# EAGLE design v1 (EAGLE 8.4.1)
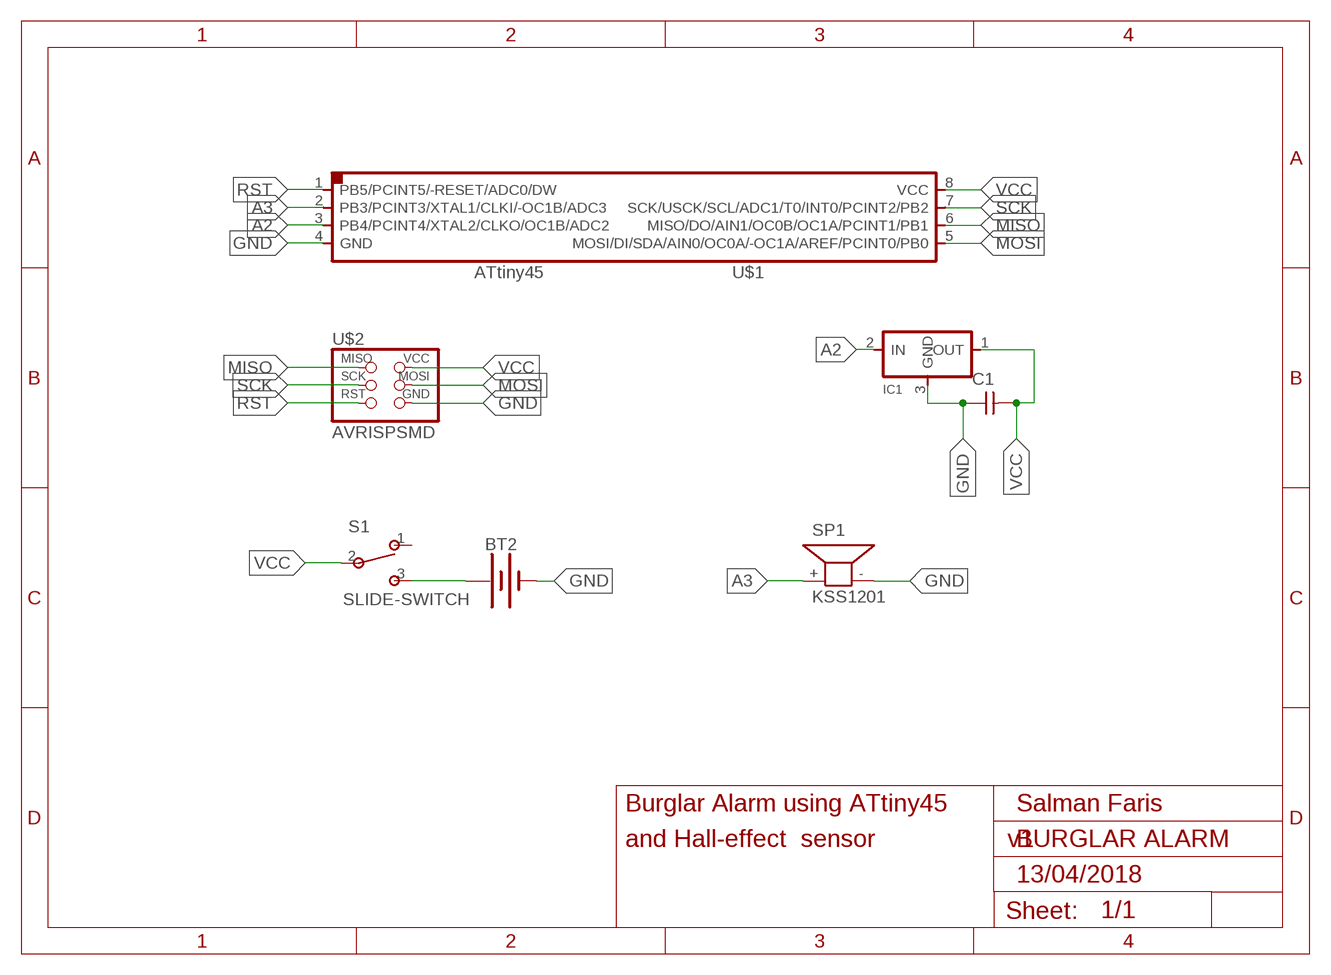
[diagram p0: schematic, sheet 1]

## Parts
BT2  BATTERY-20MM_PTH  [BATTCOM_20MM_PTH]
C1  CAP-UNPOLARIZEDFAB  [C1206FAB]
IC1  REGULATORSOT23  [SOT23]
S1  SLIDE-SWITCH  [AYZ0102AGRLC]
SP1  KSS1201  [KSS1201]
U$1  ATTINY45SI  [SOIC8]
U$2  AVRISPSMD  [2X03SMD]

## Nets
A2: IC1.2(IN) U$1.3(PB4/PCINT4/XTAL2/CLKO/OC1B/ADC2)
A3: SP1.+ U$1.2(PB3/PCINT3/XTAL1/CLKI/-OC1B/ADC3)
GND: BT2.2(-) C1.1 IC1.3(GND) SP1.- U$1.4(GND) U$2.6(GND)
MISO: U$1.6(MISO/DO/AIN1/OC0B/OC1A/PCINT1/PB1) U$2.1(MISO)
MOSI: U$1.5(MOSI/DI/SDA/AIN0/OC0A/-OC1A/AREF/PCINT0/PB0) U$2.4(MOSI)
N$1: BT2.1(+) S1.3
RST: U$1.1(PB5/PCINT5/-RESET/ADC0/DW) U$2.5(RST)
SCK: U$1.7(SCK/USCK/SCL/ADC1/T0/INT0/PCINT2/PB2) U$2.3(SCK)
VCC: C1.2 IC1.1(OUT) S1.2 U$1.8(VCC) U$2.2(VCC)
Unconnected: S1.1

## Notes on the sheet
- Burglar Alarm using ATtiny45 | Salman Faris
- and Hall-effect  sensor | BURGLAR ALARM
- 13/04/2018

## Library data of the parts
BT2 = SparkFun-Batteries:BATTERY: Battery - Single Cell; PROD_ID: BATT-09031; SF_SKU: PRT-00783
C1 = fab:CAP-UNPOLARIZED
IC1 = fab:REGULATOR
S1 = fab:SLIDE-SWITCH: SMD slide-switch AYZ0102AGRLC as found in the fablab inventory. Includes the mounting holes. Made by Zaerc.
SP1 = buzzer:KSS1201: SPEAKER
U$1 = fab:ATTINY45
U$2 = fab:AVRISP

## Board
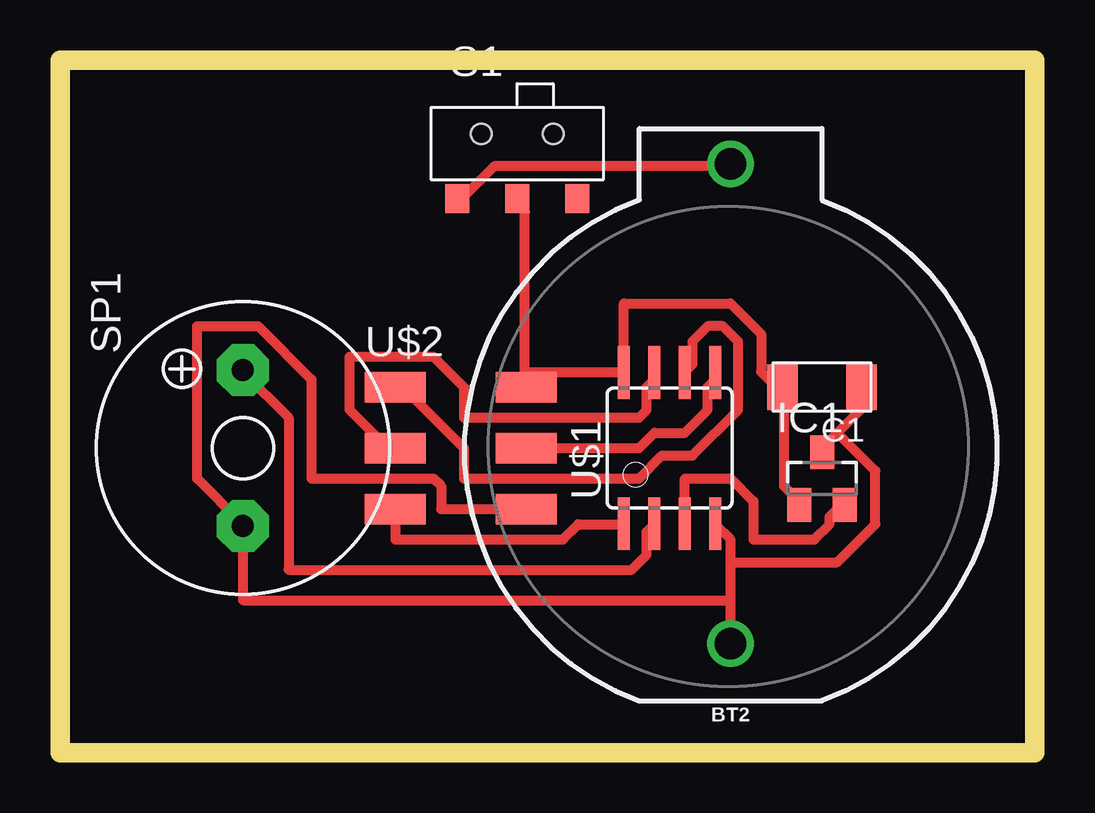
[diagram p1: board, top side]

Size 40.62 x 28.88 mm. Coordinates in mm from the lower left corner, seen from the top.
Outline: 0,0 40.62,0 40.62,28.88 0,28.88 0,0
Copper layers (1*16): Top 0.035mm / dielectric 1.5mm / Bottom 0.035mm
Design rules "default *": minimum track width 16mil, minimum drill 0.35mm, track to track 16mil, track to pad 16mil, pad to pad 16mil, via to via 16mil, smd to smd 16mil, copper to edge 16mil, drill to drill 16mil, minimum pad ring 10mil, minimum via ring 8mil, stop-mask expansion 4mil, vias tented up to drill 0mil, thermal gap 10mil

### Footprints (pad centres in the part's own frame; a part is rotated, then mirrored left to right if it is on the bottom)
BATTCOM_20MM_PTH = drill 1.3: 1 11.85,0; 2 -8.15,0
C1206FAB = smd 1.27 x 1.905: 1 -1.651,0; 2 1.651,0
SOT23 = smd 1 x 1.4: 1 -0.95,-1.1; 2 0.95,-1.1; 3 0,1.1
AYZ0102AGRLC = smd 1 x 1.2: 1 2.5,-2.3; 2 0,-2.3; 3 -2.5,-2.3 | hole 0.85: -1.5,0.4; 1.5,0.4
KSS1201 = drill 0.914 pad 2.159 octagon: + 3.251,0; - -3.251,0
SOIC8 = smd 0.5 x 2.2: 1 -1.905,-3.154; 2 -0.645,-3.154; 3 0.625,-3.154; 4 1.895,-3.154; 5 1.905,3.154; 6 0.635,3.154; 7 -0.635,3.154; 8 -1.905,3.154
2X03SMD = smd 2.54 x 1.27: 1 -2.54,2.54; 2 2.92,2.54; 3 -2.54,0; 4 2.92,0; 5 -2.54,-2.54; 6 2.92,-2.54

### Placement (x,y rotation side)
BT2  27.94,12.7 90 top
C1  31.75,15.24 180 top
IC1  31.75,11.43 0 top
S1  19.05,25.4 0 top
SP1  7.62,12.7 90 top
U$1  25.4,12.7 0 top
U$2  16.51,12.7 0 top

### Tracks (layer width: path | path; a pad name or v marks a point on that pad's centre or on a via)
A2
  Top 0.406: IC1.2 32.38,10.16 32.07,9.84 32.07,9.53 31.43,8.89 28.89,8.89 28.89,10.48 27.94,11.43 26.04,11.43 26.04,9.84 U$1.3
A3
  Top 0.406: U$1.2 24.77,9.53 24.45,9.21 24.45,8.26 23.81,7.62 9.53,7.62 9.53,13.97 7.62,15.88 SP1.+
GND
  Top 0.406: 32.38,13.34 33.34,14.29 33.34,15.24 C1.1 | 32.38,13.34 31.75,12.7 IC1.3 | BT2.2 27.94,6.35 | 27.94,6.35 27.94,7.94 | 27.94,7.94 27.94,8.89 27.3,9.53 U$1.4 | 32.38,13.34 33.97,11.75 33.97,9.53 32.38,7.94 27.94,7.94 | U$2.6 15.88,10.16 15.88,11.11 15.56,11.43 10.48,11.43 10.48,15.56 8.25,17.78 5.71,17.78 5.71,11.43 7.62,9.53 SP1.- 7.62,6.35 27.94,6.35
MISO
  Top 0.406: U$2.1 14.29,15.24 16.83,12.7 16.83,11.43 24.13,11.43 25.08,12.38 26.35,12.38 28.26,14.29 28.26,17.14 27.62,17.78 26.99,17.78 26.35,17.14 26.35,16.19 26.04,15.88 U$1.6
MOSI
  Top 0.406: U$2.4 24.13,12.7 24.77,13.34 26.04,13.34 26.99,14.29 26.99,15.24 27.3,15.56 U$1.5
N$1
  Top 0.406: S1.3 16.83,23.18 18.1,24.45 27.94,24.45 BT2.1
RST
  Top 0.406: U$2.5 13.97,8.89 20.95,8.89 21.59,9.53 23.49,9.53 U$1.1
SCK
  Top 0.406: U$2.3 13.65,12.7 12.06,14.29 12.06,16.51 15.56,16.51 16.83,15.24 16.83,13.97 24.13,13.97 24.45,14.29 24.45,15.24 24.77,15.56 U$1.7
VCC
  Top 0.406: IC1.1 30.8,10.48 30.16,11.11 30.16,15.24 C1.2 29.84,15.24 29.21,15.88 29.21,17.46 27.94,18.73 23.49,18.73 23.49,15.88 | 19.37,15.88 19.37,15.24 U$2.2 | 19.37,15.88 19.37,22.54 19.05,22.86 S1.2 | 19.37,15.88 23.49,15.88 | 23.49,15.88 U$1.8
